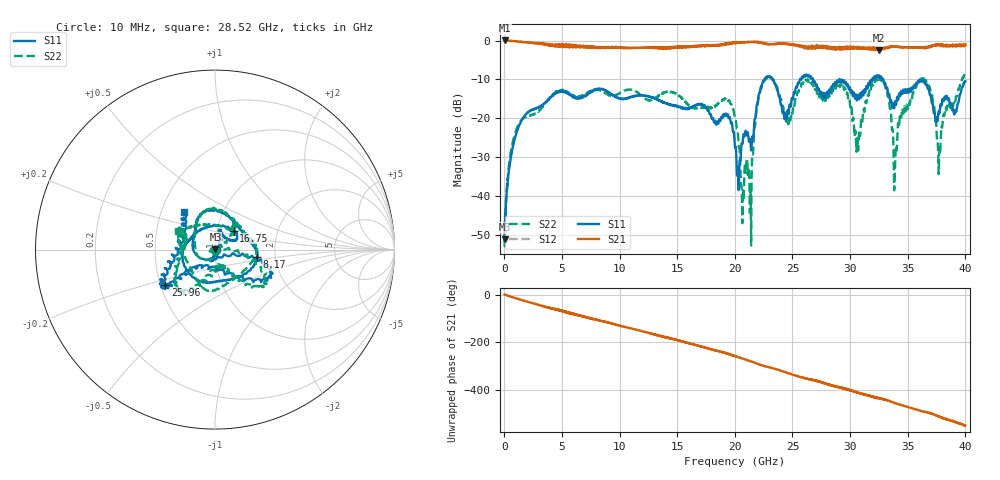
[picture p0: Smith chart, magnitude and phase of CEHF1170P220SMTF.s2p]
!Agilent Technologies,N5224A,MY51441447,A.10.00.00
!Agilent N5224A: A.10.00.00
!Date: Wednesday, January 15, 2020 16:43:17
!Correction: S11(Full 2 Port(1,2))
!S21(Full 2 Port(1,2))
!S12(Full 2 Port(1,2))
!S22(Full 2 Port(1,2))
!S2P File: Measurements: S11, S21, S12, S22:
# Hz S  dB  R 50
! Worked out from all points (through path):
!   4001 points, 10 MHz to 40.01 GHz, reference 50 ohm
!   highest |S21| = 0.02 dB at 10 MHz (marker M1); lowest = -2.4 dB at 32.52 GHz (marker M2)
!   group delay of S21, straight-line fit = 37.5 ps
!   lowest |S11| = -51.2 dB at 20 MHz (marker M3), VSWR 1.01, Z = 50.3 + j0.0632 ohm
!   |S11| at or under -10 dB: start of sweep to 22.57 GHz; 29.08 GHz to 31.93 GHz (2.849 GHz wide, 9.34 % of centre); 32.88 GHz to end of sweep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
!   |S22| runs from -53.0 to -8.5 dB; largest |S21 - S12| = 0.099
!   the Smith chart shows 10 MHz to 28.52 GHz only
!   S11 on the Smith chart (normalised r, x): 10 MHz: 1.01, -0.00; 8.17 GHz: 1.60, -0.15; 16.75 GHz: 1.20, +0.26; 25.96 GHz: 0.53, -0.24; 28.52 GHz: 0.65, +0.29
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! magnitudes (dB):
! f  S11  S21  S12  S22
! 10 MHz  -50.4  0.0  0.0  -47.6
! 20 MHz  -51.2  0.0  0.0  -53.0
! 1.6 GHz  -19.9  -0.4  -0.4  -20.0
! 6.68 GHz  -14.7  -1.7  -1.6  -14.3
! 8.17 GHz  -12.5  -1.9  -1.7  -12.8
! 13.35 GHz  -15.4  -1.7  -2.0  -14.3
! 16.75 GHz  -16.6  -1.4  -1.3  -17.4
! 20.01 GHz  -27.4  -0.5  -0.6  -19.6
! 20.62 GHz  -26.5  -0.5  -0.5  -41.6
! 21.28 GHz  -25.5  -0.4  -0.4  -41.2
! 22.55 GHz  -10.2  -0.7  -0.8  -10.3
! 24.63 GHz  -18.7  -1.0  -0.9  -21.5
! 25.96 GHz  -9.4  -1.6  -2.0  -10.5
! 26.68 GHz  -10.0  -2.0  -1.7  -10.8
! 28.52 GHz  -11.3  -2.0  -2.0  -12.6
! 30.69 GHz  -14.0  -2.0  -2.0  -28.0
! 32.52 GHz  -9.1  -2.4  -2.2  -10.1
! 33.35 GHz  -13.9  -1.7  -1.7  -14.5
! 33.92 GHz  -15.6  -1.6  -1.5  -30.4
! 36.55 GHz  -11.3  -1.8  -1.8  -10.1
! 37.71 GHz  -18.4  -1.0  -1.1  -32.3
! 40.01 GHz  -10.5  -1.0  -1.5  -8.7
